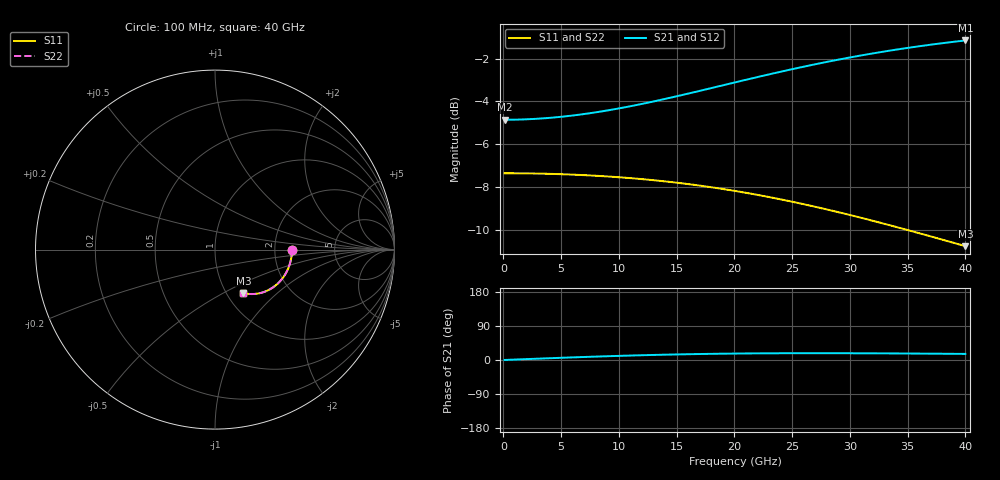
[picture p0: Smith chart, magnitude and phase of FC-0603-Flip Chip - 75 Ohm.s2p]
!Vishay Thin-Film
!FC Family
!Case Size 0603
!Assembly Style Flip Chip
!11/9/2015
!thinfilm@vishay.com
# GHz S MA R 50
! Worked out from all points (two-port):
!   101 points, 100 MHz to 40 GHz, reference 50 ohm
!   highest |S21| = -1.15 dB at 40 GHz (marker M1); lowest = -4.9 dB at 100 MHz (marker M2)
!   |S21| within 3 dB of the highest: 11.68 GHz to end of sweep
!   lowest |S11| = -10.8 dB at 40 GHz (marker M3), VSWR 1.81, Z = 59.7 - j31.6 ohm
!   |S11| at or under -10 dB: 34.89 GHz to end of sweep
!   |S22| runs from -10.8 to -7.4 dB; largest |S21 - S12| = 0
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0.1  0.4286 -0.2  0.5714 0.1  0.5714 0.1  0.4286 -0.2
1.696  0.4283 -2.7  0.5725 2.0  0.5725 2.0  0.4283 -2.7
3.292  0.4276 -5.2  0.5755 3.9  0.5755 3.9  0.4276 -5.2
4.888  0.4264 -7.7  0.5803 5.7  0.5803 5.7  0.4264 -7.7
6.883  0.4243 -10.9  0.5889 7.8  0.5889 7.8  0.4243 -10.9
8.479  0.4221 -13.5  0.5976 9.5  0.5976 9.5  0.4221 -13.5
10.075  0.4193 -16.0  0.608 11.0  0.608 11.0  0.4193 -16.0
11.671  0.416 -18.5  0.6198 12.3  0.6198 12.3  0.416 -18.5
13.666  0.4111 -21.7  0.6364 13.8  0.6364 13.8  0.4111 -21.7
16.858  0.4014 -26.7  0.6663 15.7  0.6663 15.7  0.4014 -26.7
18.454  0.3958 -29.2  0.6823 16.4  0.6823 16.4  0.3958 -29.2
20.05  0.3896 -31.6  0.6987 17.0  0.6987 17.0  0.3896 -31.6
21.646  0.383 -34.0  0.7154 17.4  0.7154 17.4  0.383 -34.0
23.242  0.3759 -36.4  0.7321 17.7  0.7321 17.7  0.3759 -36.4
24.838  0.3684 -38.7  0.7486 17.9  0.7486 17.9  0.3684 -38.7
26.833  0.3586 -41.4  0.7687 18.0  0.7687 18.0  0.3586 -41.4
28.429  0.3505 -43.6  0.7843 17.9  0.7843 17.9  0.3505 -43.6
30.025  0.3422 -45.7  0.7993 17.8  0.7993 17.8  0.3422 -45.7
31.621  0.3337 -47.7  0.8135 17.7  0.8135 17.7  0.3337 -47.7
33.616  0.3231 -50.0  0.8303 17.4  0.8303 17.4  0.3231 -50.0
36.808  0.3061 -53.6  0.8546 16.8  0.8546 16.8  0.3061 -53.6
40  0.2894 -56.8  0.8757 16.1  0.8757 16.1  0.2894 -56.8
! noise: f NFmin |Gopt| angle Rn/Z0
0.1  -1.929e-15  1  -1.207e-06  1.5
4.489  -4.822e-16  1  -8.538e-07  1.44
8.878  1.929e-15  1  8.6e-15  1.284
13.27  -1.446e-15  1  -1.207e-06  1.072
17.66  7.782e-08  1  2.057e-15  0.8503
22.05  0  1  7.081e-15  0.6507
26.43  0  1  -1.708e-06  0.4875
30.82  -4.822e-16  1  -8.538e-07  0.3618
35.21  2.456e-08  1  0  0.2684
40  2.522e-08  1  7.983e-14  0.1948
